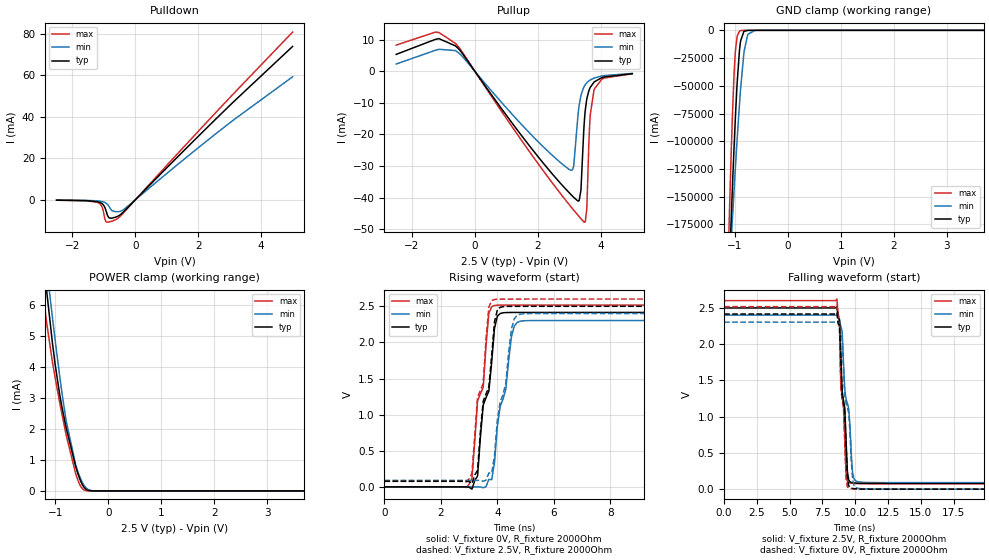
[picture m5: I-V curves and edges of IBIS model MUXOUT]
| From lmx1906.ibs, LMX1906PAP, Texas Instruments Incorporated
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|   Model MUXOUT
[Model]   MUXOUT
Model_type   Output
Polarity   Non-Inverting
Vmeas = 1.25
Vref = 1.25
Cref = 2pF
Rref = 50
|   typ   min   max
C_comp   0.717pF   0.704pF   0.730pF
[Voltage Range]   2.5   2.4   2.6
[Temperature Range]   27   105   -40
[Pullup Reference]   2.5   2.4   2.6
[Pulldown Reference]   0   0   0
[Power Clamp Reference]   2.5   2.4   2.6
[GND Clamp Reference]   0   0   0
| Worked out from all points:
|   slope of the pulldown table from 0 to 0.375 V, typ, clamps not added: 64.6 ohm
|   slope of the pullup table from 0 to 0.375 V, typ, clamps not added: 70.7 ohm
|   GND clamp passes 1 mA (typ) near -0.53 V on its own axis
|   POWER clamp passes 1 mA (typ) near -0.65 V on its own axis
|   falling waveform, V_fixture 2.5V, R_fixture 2000Ohm: 20-80 % time 457ps typ, 623ps min, 404ps max; typ from 2.5 V to 0.078 V
|   rising waveform, V_fixture 0V, R_fixture 2000Ohm: 20-80 % time 482ps typ, 504ps min, 436ps max; typ from 0 V to 2.42 V
|   rising waveform, V_fixture 2.5V, R_fixture 2000Ohm: 20-80 % time 480ps typ, 500ps min, 434ps max; typ from 0.078 V to 2.5 V
|   falling waveform, V_fixture 0V, R_fixture 2000Ohm: 20-80 % time 456ps typ, 621ps min, 403ps max; typ from 2.42 V to 0 V
[Pulldown]
|   Voltage   I(typ)   I(min)   I(max)
-2.5V     -152.1uA   -105.3uA   -156.9uA
-1.218V   -863.2uA   -483uA     -1.124mA
-1.06V    -1.767mA   -801.7uA   -3.259mA
-962.5mV  -3.78mA    -1.277mA   -9.353mA
-925mV    -5.414mA   -1.607mA   -10.58mA
-880mV    -7.565mA   -2.212mA   -10.74mA
-827.5mV  -8.685mA   -3.325mA   -10.6mA
-737.5mV  -8.773mA   -5.213mA   -10.24mA
-565mV    -7.976mA   -5.698mA   -9.035mA
-340mV    -5.27mA    -4.327mA   -5.657mA
2.638V    40.06mA    32.74mA    43.3mA
5V        73.87mA    59.25mA    80.77mA
[GND Clamp]
|   Voltage   I(typ)   I(min)   I(max)
-2.5V     -2.29kA    -1.568kA   -2.957kA
-1.143V   -269.9A    -256.8A    -237A
-1.067V   -171.7A    -190.8A    -112.2A
-1.045V   -143.9A    -171.6A    -79.67A
-1.015V   -108.6A    -146.5A    -43.02A
-985mV    -76.29A    -122.2A    -17.71A
-955mV    -48.2A     -98.87A    -5.358A
-910mV    -17.98A    -66.5A     -651.3mA
-820mV    -859.4mA   -18.23A    -17.1mA
-752.5mV  -71.62mA   -3.59A     -6.741mA
-617.5mV  -3.365mA   -67.05mA   -1.684mA
5V        0A         0A         0A
[Pullup]
|   Voltage   I(typ)   I(min)   I(max)
-2.5V     5.389mA    2.339mA    8.327mA
-1.255V   10.15mA    6.685mA    12.45mA
-617.5mV  8.072mA    6.59mA     8.855mA
3.058V    -39.11mA   -31.37mA   -43mA
3.14V     -39.94mA   -29.85mA   -44mA
3.312V    -40.94mA   -10.69mA   -46.05mA
3.373V    -36.86mA   -7.467mA   -46.74mA
3.485V    -14.72mA   -4.557mA   -47.81mA
3.553V    -8.902mA   -3.65mA    -43.74mA
3.665V    -5.066mA   -2.721mA   -13.76mA
3.785V    -3.398mA   -2.129mA   -5.84mA
5V        -748.2uA   -648.3uA   -750.2uA
[POWER Clamp]
|   Voltage   I(typ)   I(min)   I(max)
-2.5V     43.77mA    42.57mA    41.7mA
-1.337V   9.384mA    9.933mA    8.082mA
-1.173V   6.575mA    7.331mA    5.521mA
-1.06V    4.839mA    5.66mA     4.207mA
-1V       4.03mA     4.804mA    3.61mA
-880mV    2.742mA    3.213mA    2.511mA
-797.5mV  2.045mA    2.271mA    1.817mA
-617.5mV  793.5uA    852.7uA    560.8uA
-535mV    369.3uA    442.3uA    189uA
-452.5mV  105.1uA    166.3uA    27.34uA
-242.5mV  289.3nA    1.905uA    1.867nA
5V        0A         0A         0A
[Ramp]
R_load = 2000
|   typ   min   max
dV/dt_r   1.44911/4.8168e-10   1.38188/5.04235e-10   1.51025/4.36096e-10
dV/dt_f   1.45316/4.57295e-10   1.38595/6.22846e-10   1.51447/4.03675e-10
[Falling Waveform]
V_fixture = 2.5V
V_fixture_min = 2.4V
V_fixture_max = 2.6V
R_fixture = 2000Ohm
C_fixture = 0F
|   Time   V(typ)   V(min)   V(max)
0s        2.5V       2.4V       2.6V
8.6ns     2.519V     2.4V       2.622V
8.8ns     2.342V     2.318V     2.303V
8.9ns     1.866V     2.247V     1.452V
9ns       1.351V     2.176V     1.27V
9.3ns     671.8mV    1.241V     215.9mV
9.5ns     127.3mV    1.114V     91.07mV
9.8ns     88.17mV    227.1mV    80.67mV
10.1ns    82.22mV    107.8mV    77.63mV
24.9ns    78.06mV    90.08mV    75.88mV
[Rising Waveform]
V_fixture = 0V
V_fixture_min = 0V
V_fixture_max = 0V
R_fixture = 2000Ohm
C_fixture = 0F
|   Time   V(typ)   V(min)   V(max)
0s        -28.96nV   112.5nV    -62.28nV
3ns       -4.718mV   -748.2nV   37.26mV
3.1ns     -31.66mV   738.8nV    113.9mV
3.3ns     150.9mV    42.97uV    1.193V
3.5ns     1.133V     -12.77mV   1.378V
3.7ns     1.327V     103.9mV    2.405V
3.9ns     2.195V     335.8mV    2.511V
4.5ns     2.414V     2.079V     2.517V
4.8ns     2.415V     2.292V     2.517V
24.9ns    2.415V     2.303V     2.517V
[Rising Waveform]
V_fixture = 2.5V
V_fixture_min = 2.4V
V_fixture_max = 2.6V
R_fixture = 2000Ohm
C_fixture = 0F
|   Time   V(typ)   V(min)   V(max)
0s        78.06mV    90.08mV    75.88mV
3ns       73.28mV    90.08mV    112.8mV
3.1ns     45.72mV    90.08mV    185.7mV
3.3ns     231mV      90.13mV    1.243V
3.5ns     1.187V     77.08mV    1.432V
3.7ns     1.383V     192mV      2.491V
3.9ns     2.287V     431.4mV    2.594V
4.5ns     2.499V     2.186V     2.6V
4.8ns     2.5V       2.39V      2.6V
24.9ns    2.5V       2.4V       2.6V
[Falling Waveform]
|Gnd
V_fixture = 0V
V_fixture_min = 0V
V_fixture_max = 0V
R_fixture = 2000Ohm
C_fixture = 0F
|   Time   V(typ)   V(min)   V(max)
0s        2.415V     2.303V     2.517V
8.6ns     2.434V     2.303V     2.538V
8.8ns     2.265V     2.223V     2.228V
8.9ns     1.791V     2.157V     1.399V
9ns       1.299V     2.088V     1.223V
9.3ns     594.6mV    1.183V     139.5mV
9.5ns     48.4mV     1.053V     14.86mV
9.8ns     9.816mV    135.2mV    4.703mV
10.1ns    4.063mV    17mV       1.731mV
24.9ns    -28.96nV   112.5nV    -62.25nV
